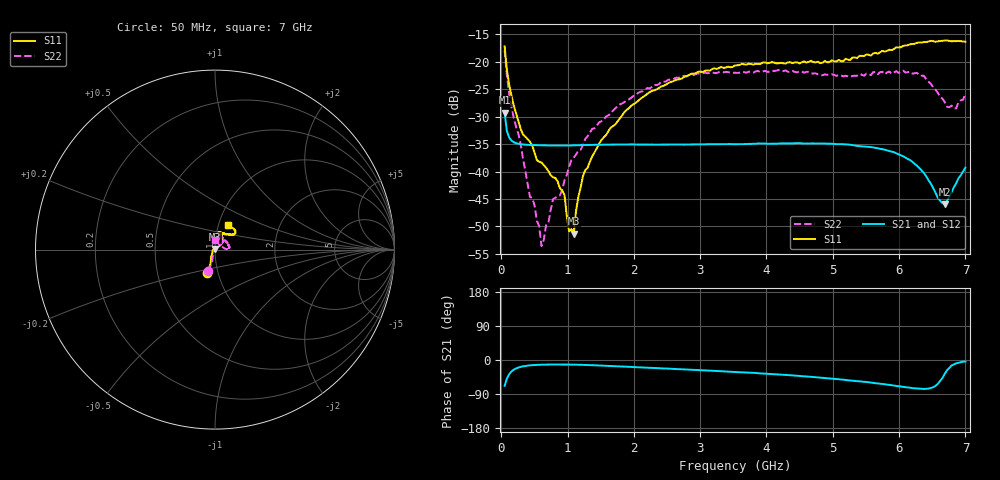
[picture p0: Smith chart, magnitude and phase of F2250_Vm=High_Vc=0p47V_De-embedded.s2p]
! Integrated Device Technology
! Corporate Headquarters
! 6024 Silver Creek Valley Road
! San Jose, CA 95138  USA
! Phone:  1-408-284-8200
! Toll Free:  1-800-223-1366
! Webpage:  http://www.idt.com/
! Timing and RF Division
! 515 Groton Road, Suite 102
! Westford, MA 01886-6024
! Device:  F2250
! Description: Voltage Variable RF Attenuator
! Frequency:  50.0 -  6000.00 MHz
! Package:  3x3 mm Thin QFN Plastic Package: 16 pin
! Ports:  2 RF, 3 DC
!  Pin  1  = GND
!  Pin  2  = NC
!  Pin  3  = RF1  = Port 1
!  Pin  4  = NC
!  Pin  5  = GND
!  Pin  6  = GND
!  Pin  7  = GND
!  Pin  8  = GND
!  Pin  9  = NC
!  Pin 10  = RF2  = Port 2
!  Pin 11  = NC
!  Pin 12  = GND
!  Pin 13  = GND
!  Pin 14  = VCNTRL
!  Pin 15  = VDD
!  Pin 16  = VMODE
! Vcntrl:  0.470 Volts
! Vmode:  +3.300 Volts
! Vdd:  +3.30  Volts
! Current:  1.266 mA
! Data:  The device was measured on a the F2250 evaluation board which has
!  individual transmission lines to the RF pins.  Data was collected
!  using a calibrated network analyzer.  The evaluation board was
!  de-embedded using a TRL calibration technique.
!  The reference plane is the edge of the package pin.
! Misc:  SN 10
!  Action Tracker AT0258
! Date Measured:  2014-11-26
! Date:  2015-10-15  MJV
! Note:
!  Integrated Device Technology supplies this data as a sample of measured
!  data at the package pin for this product.  Your particular data for this
!  product may vary.
!  Data was taken at 25 degrees C.
!  Integrated Device Technology reserves the right to change this data at anytime.
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# GHz S dB R 50
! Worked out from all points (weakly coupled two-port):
!   201 points, 50 MHz to 7 GHz, reference 50 ohm
!   highest |S21| = -29.26 dB at 50 MHz (marker M1); lowest = -46.0 dB at 6.687 GHz (marker M2)
!   lowest |S11| = -51.3 dB at 1.093 GHz (marker M3), VSWR 1.01, Z = 50 + j0.271 ohm
!   |S11| at or under -10 dB: start of sweep to end of sweep
!   |S22| runs from -53.6 to -17.8 dB; largest |S21 - S12| = 5.1e-05
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0.05  -17.17 -108.5  -29.26 -68.1  -29.26 -68.1  -17.83 -108.3
0.1195  -24.20 -111.9  -33.83 -37.3  -33.83 -37.3  -25.88 -105.7
0.29325  -32.26 -127.2  -35.01 -18.1  -35.01 -18.1  -35.04 -109.6
0.43225  -34.57 -145.2  -35.16 -14.1  -35.16 -14.1  -44.63 -138.9
0.57125  -38.22 -161.2  -35.22 -12.6  -35.22 -12.6  -49.94 -178.0
0.606  -38.37 -162.3  -35.23 -12.4  -35.22 -12.4  -53.61 161.6
0.77975  -41.05 176.4  -35.25 -11.9  -35.25 -11.9  -45.05 87.1
0.884  -43.05 165.3  -35.25 -11.9  -35.25 -11.9  -44.35 71.7
0.9535  -44.30 170.7  -35.26 -12.0  -35.26 -12.0  -41.56 73.2
1.023  -50.92 140.6  -35.24 -12.1  -35.25 -12.1  -39.15 60.1
1.0925  -51.33 89.0  -35.23 -12.3  -35.23 -12.3  -37.48 56.8
1.12725  -47.22 60.7  -35.22 -12.4  -35.22 -12.4  -36.90 50.8
1.2315  -40.85 40.2  -35.18 -12.8  -35.19 -12.8  -35.17 42.6
1.6485  -32.03 40.9  -35.11 -15.6  -35.11 -15.6  -29.45 42.9
2.37825  -24.75 46.6  -35.08 -21.6  -35.08 -21.7  -24.07 44.8
3.525  -20.65 71.6  -35.01 -31.5  -35.02 -31.5  -21.97 68.1
4.7065  -20.06 72.0  -34.88 -44.9  -34.87 -44.9  -22.13 67.5
5.85325  -17.79 40.5  -36.26 -65.7  -36.27 -65.8  -21.76 18.8
6.3745  -16.40 40.9  -40.26 -76.4  -40.28 -76.5  -22.55 2.4
6.68725  -16.12 47.8  -46.00 -36.9  -46.01 -36.6  -27.30 24.5
6.861  -16.22 54.5  -42.14 -8.8  -42.11 -8.9  -28.50 58.4
7  -16.33 62.4  -39.28 -4.1  -39.26 -4.3  -25.77 87.7
